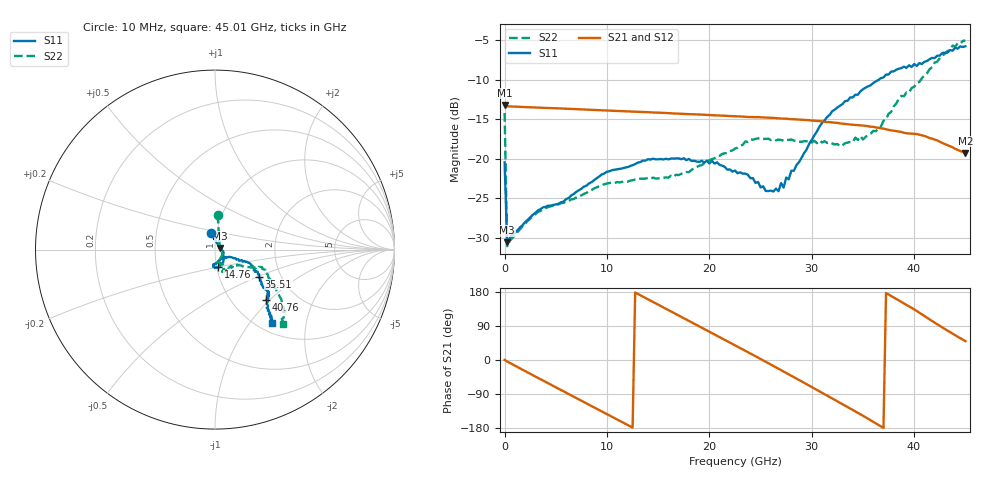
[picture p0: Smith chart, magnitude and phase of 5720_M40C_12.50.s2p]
! Device:  ADRF5720
! Description: 0.5dB LSB GaAs MMIC 6-bit Digital Attenuator
! Frequency:  0.000009 -  40 GHz
! Ports:
!	RF1	= Port 1
!	RF2	= Port 2
! Vdd:  3.3 Volt
! Vss:  -3.3 Volt
! Control:  0/3.3 Volt
! State:  12.50 dB attenuation
! Data:  The device was measured using G-S-G Probes on a matrix board.
!  Data was collected using an calibrated 4 port network analyzer.
!  The reference plane for this measurement is at the launchers.
! Note:  Analog Devices supplies this data as a sample of measured data
!  for this product.  Your particular data for this product may vary.
!  Data was taken at -40 degrees C.
!  Analog Devices reserves the right to change this data at anytime.
# GHZ S DB R 45.0
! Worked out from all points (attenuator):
!   181 points, 10 MHz to 45.01 GHz, reference 45 ohm
!   highest |S21| = -13.18 dB at 10 MHz (marker M1); lowest = -19.3 dB at 45.01 GHz (marker M2)
!   lowest |S11| = -30.6 dB at 260 MHz (marker M3), VSWR 1.06, Z = 47.6 + j0.81 ohm
!   |S11| at or under -10 dB: start of sweep to 36.53 GHz
!   |S22| runs from -31.1 to -5.0 dB; largest |S21 - S12| = 0.00081
!   S11 on the Smith chart (normalised r, x): 10 MHz: 0.94, +0.17; 14.76 GHz: 1.02, -0.20; 35.51 GHz: 1.55, -0.51; 40.76 GHz: 1.42, -0.95; 45.01 GHz: 1.16, -1.29
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0.01  -20.47 104.4  -13.18 0.2  -13.20 0.2  -14.21 85.7
0.26  -30.60 16.7  -13.36 -3.9  -13.38 -4.0  -31.09 15.5
3.26  -26.56 -13.4  -13.52 -47.1  -13.55 -47.2  -26.77 -27.7
5.51  -25.52 -27.7  -13.64 -79.2  -13.66 -79.2  -25.65 -45.1
7.76  -23.54 -44.0  -13.76 -111.1  -13.78 -111.1  -24.46 -61.5
11.26  -21.29 -61.9  -13.96 -160.7  -13.98 -160.7  -23.01 -73.8
14.76  -20.08 -79.5  -14.15 149.6  -14.17 149.5  -22.52 -75.8
15.26  -20.04 -81.5  -14.17 142.4  -14.19 142.3  -22.48 -75.3
19.01  -20.40 -92.8  -14.40 88.9  -14.42 88.8  -20.89 -64.5
20.76  -20.46 -93.4  -14.51 63.8  -14.53 63.8  -19.68 -62.1
22.76  -21.84 -95.2  -14.64 35.1  -14.66 35.0  -18.62 -65.9
24.01  -22.47 -84.0  -14.72 17.2  -14.74 17.1  -17.56 -67.0
25.51  -24.09 -65.1  -14.79 -4.8  -14.81 -5.0  -17.49 -68.2
26.76  -24.12 -46.3  -14.89 -23.1  -14.91 -23.3  -17.57 -69.3
30.26  -17.04 -22.2  -15.18 -75.2  -15.21 -75.3  -17.72 -69.0
32.76  -13.29 -22.5  -15.52 -113.0  -15.54 -113.1  -18.42 -57.7
35.51  -10.83 -31.7  -15.89 -155.2  -15.91 -155.4  -16.99 -37.4
37.76  -8.96 -38.4  -16.41 169.1  -16.43 168.9  -14.07 -28.9
38.76  -8.52 -37.8  -16.62 153.4  -16.65 153.1  -12.04 -24.3
40.76  -7.99 -44.5  -17.04 120.5  -17.07 120.3  -9.80 -25.1
43.76  -6.30 -49.6  -18.56 69.5  -18.58 69.2  -5.66 -41.5
45.01  -5.75 -52.1  -19.26 49.8  -19.28 49.6  -5.01 -47.5
